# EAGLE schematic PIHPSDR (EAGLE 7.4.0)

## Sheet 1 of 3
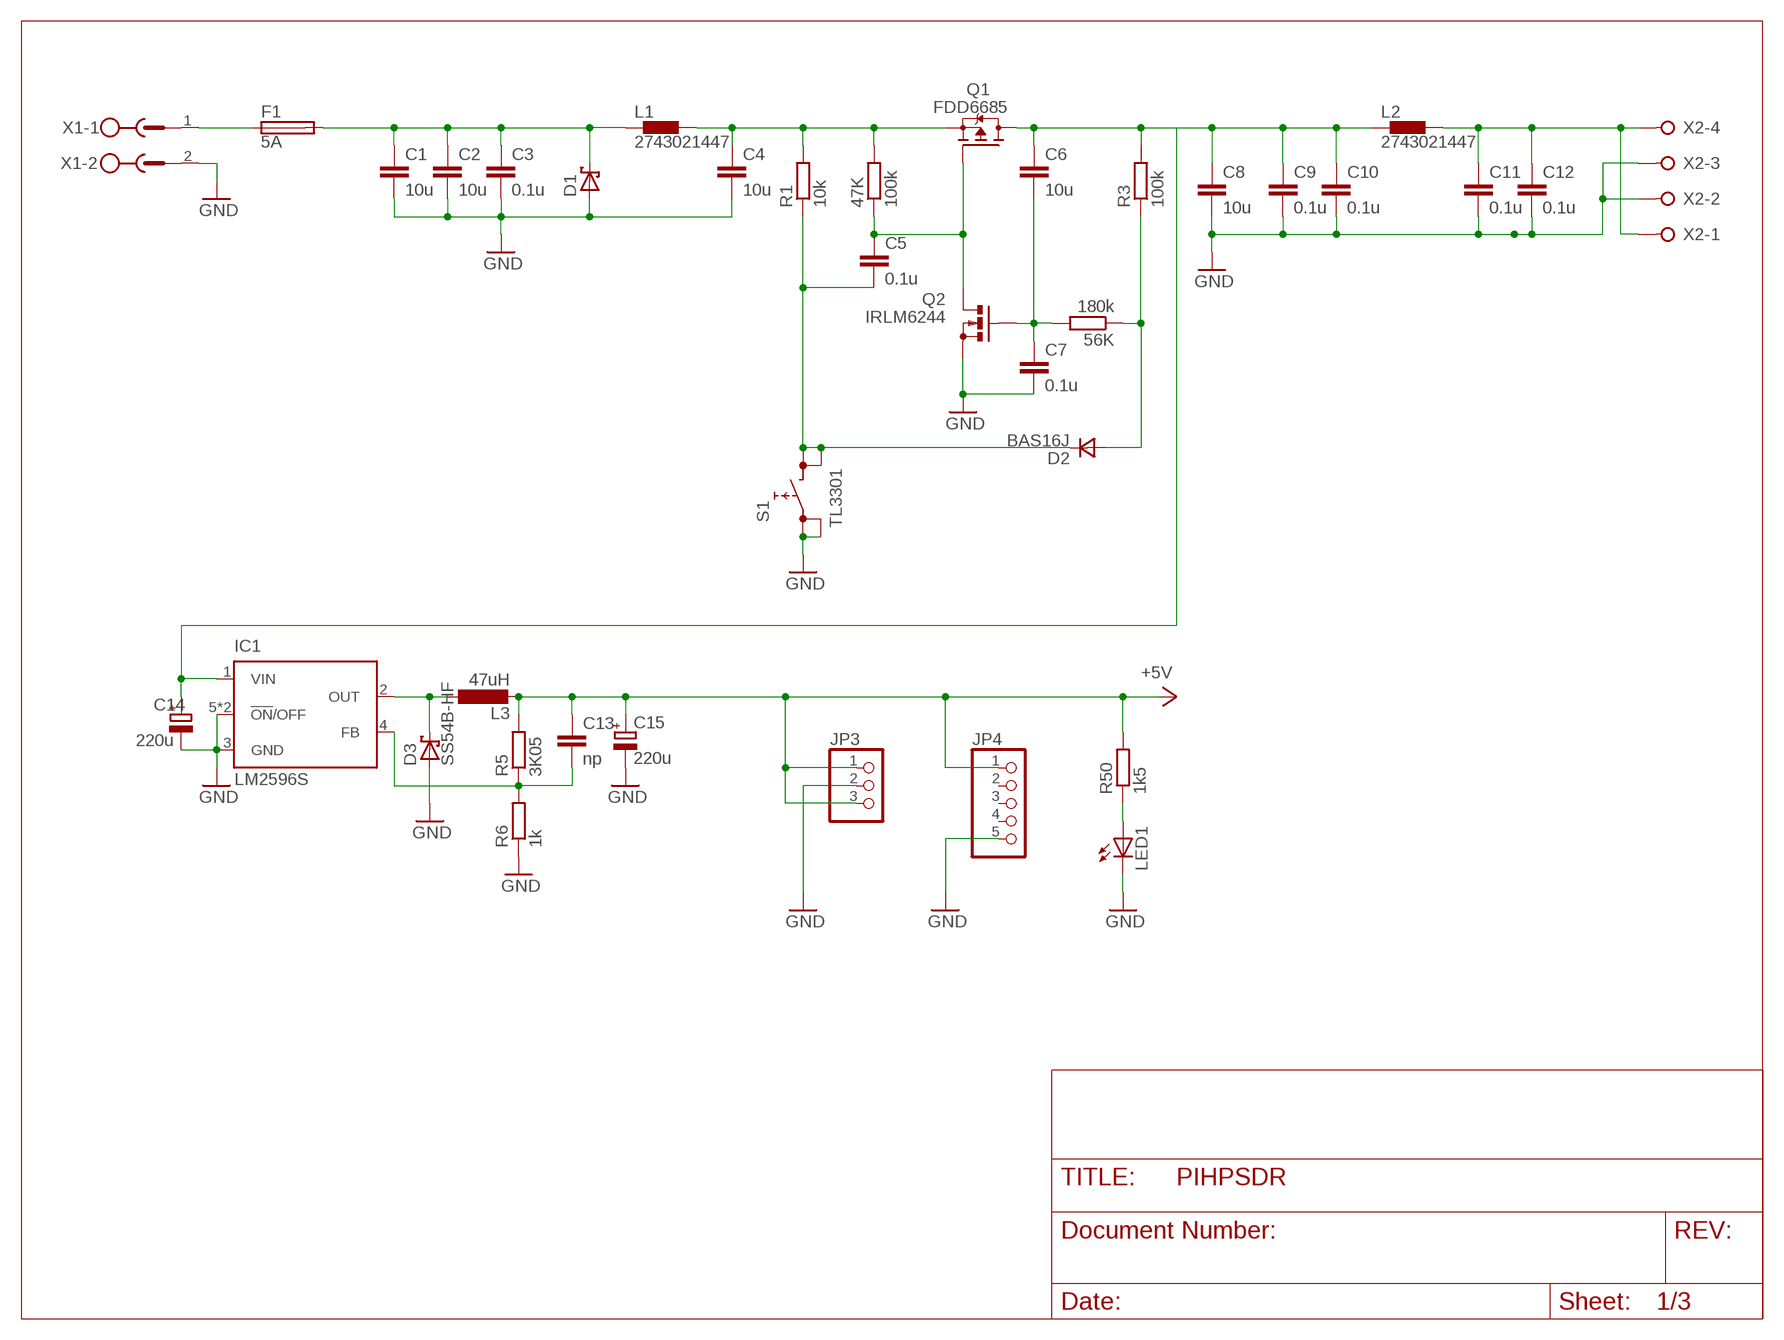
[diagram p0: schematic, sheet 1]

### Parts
47K  100k  R-EU_R0805  [R0805]
56K  180k  R-EU_R0805  [R0805]
C1  10u  C-EUC0805K  [C0805K]
C2  10u  C-EUC0805K  [C0805K]
C3  0.1u  C-EUC0805K  [C0805K]
C4  10u  C-EUC0805K  [C0805K]
C5  0.1u  C-EUC0805K  [C0805K]
C6  10u  C-EUC0805K  [C0805K]
C7  0.1u  C-EUC0805K  [C0805K]
C8  10u  C-EUC0805K  [C0805K]
C9  0.1u  C-EUC0805K  [C0805K]
C10  0.1u  C-EUC0805K  [C0805K]
C11  0.1u  C-EUC0805K  [C0805K]
C12  0.1u  C-EUC0805K  [C0805K]
C13  np  C-EUC0805  [C0805]
C14  220u  CPOL-EU140CLH-1010  [140CLH-1010]
C15  220u  CPOL-EU140CLH-1010  [140CLH-1010]
D1  SCHOTTKY-DIODESMC  [SMC]
D2  BAS16J  DSOD323  [SOD323]
D3  SS54B-HF  SCHOTTKY-DIODESMD  [SMB]
F1  5A  FUSESHK20L  [SHK20L]
IC1  LM2596S  [TO263-5]
JP3  PINHD-1X3  [1X03]
JP4  PINHD-1X5  [1X05]
L1  2743021447  [SM_BEAD]
L2  2743021447  [SM_BEAD]
L3  47uH  PULSE_PA4342  [PULSE_PA4342]
LED1  LED5MM  [LED5MM]
Q1  FDD6685  FDD4141TO252  [TO252]
Q2  IRLM6244  BS170_SMD  [SOT23]
R1  10k  R-EU_R0805  [R0805]
R3  100k  R-EU_R0805  [R0805]
R5  3K05  R-EU_R0805  [R0805]
R6  1k  R-EU_R0805  [R0805]
R50  1k5  R-EU_R0805  [R0805]
S1  TL3301  [TL3301-SMD]
X1  MSTBV2  [MSTBV2]
X2  W237-04P  [W237-4P]

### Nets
+5V: C13.1 C15.+ JP3.1 JP3.3 JP4.1 L3.2 R5.2 R50.2 ; also sheet 2,3
GND: C1.2 C2.2 C3.2 C4.2 C7.2 C8.2 C9.2 C10.2 C11.2 C12.2 C14.- C15.- D1.A D3.A IC1.3(GND) IC1.5(!ON!/OFF) IC1.6(!ON!/OFF) JP3.2 JP4.5 LED1.K(C) Q2.2(S) R6.1 S1.1 S1.2 X1.2 X2.2 X2.3 ; also sheet 2,3
N$1: F1.1A X1.1
N$2: C1.1 C2.1 C3.1 D1.C F1.2A L1.P$1
N$3: 47K.2 C4.1 L1.P$2 Q1.2(S) R1.2
N$4: 47K.1 C5.1 Q1.1(G) Q2.3(D)
N$5: C6.1 C8.1 C9.1 C10.1 C14.+ IC1.1(VIN) L2.P$1 Q1.3(D) R3.2
N$6: C5.2 D2.1(C) R1.1 S1.3 S1.4
N$7: 56K.2 C6.2 C7.1 Q2.1(G)
N$8: 56K.1 D2.2(A) R3.1
N$9: C11.1 C12.1 L2.P$2 X2.1 X2.4
N$10: D3.C IC1.2(OUT) L3.1
N$11: C13.2 IC1.4(FB) R5.1 R6.2
N$14: LED1.A R50.1
Unconnected: JP4.2 JP4.3 JP4.4

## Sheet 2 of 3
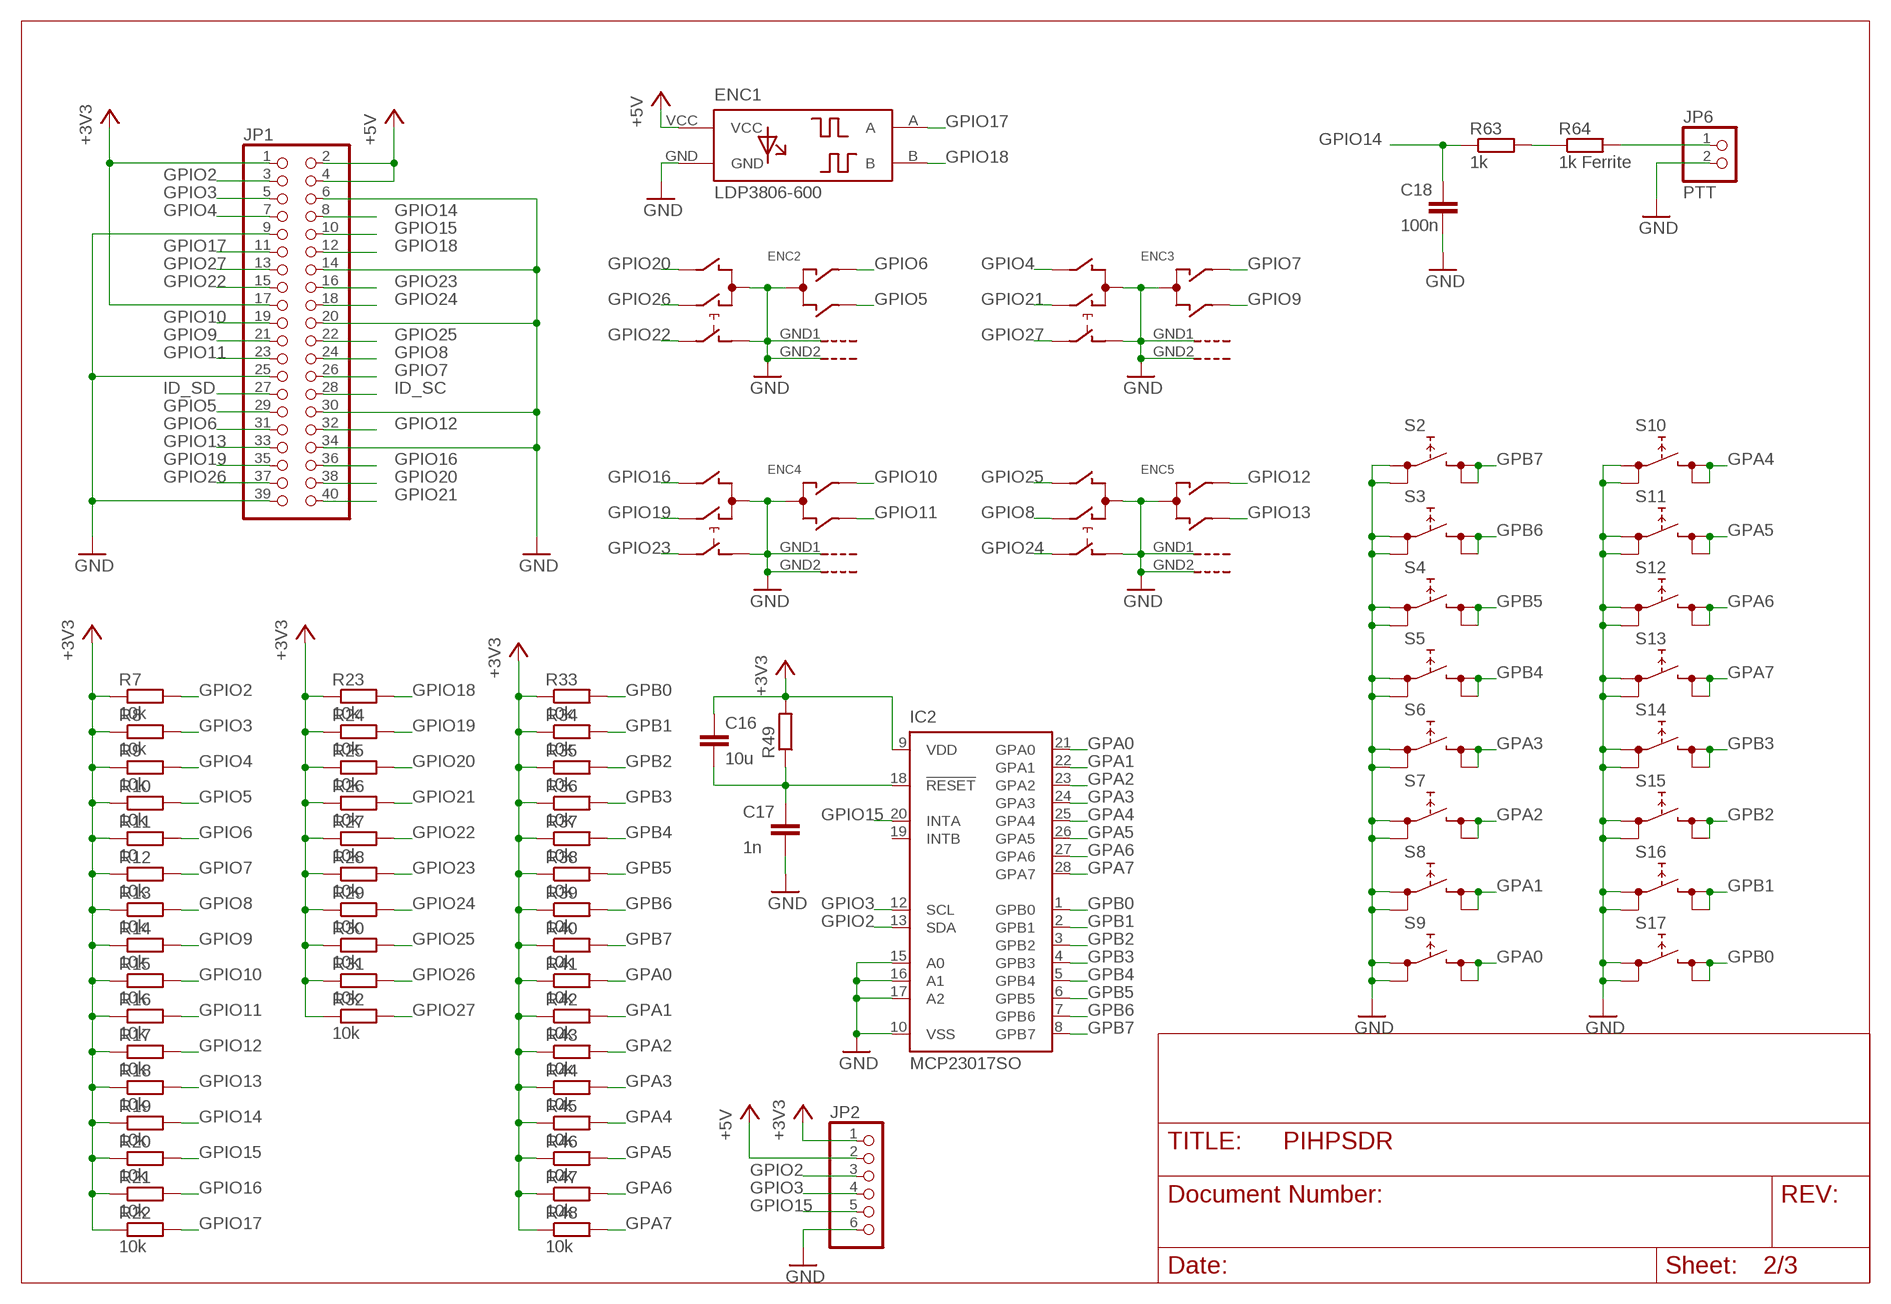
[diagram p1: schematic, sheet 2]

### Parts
C16  10u  C-EUC0805K  [C0805K]
C17  1n  C-EUC0805K  [C0805K]
C18  100n  C-EUC0805K  [C0805K]
ENC1  LDP3806-600  [LPD3806_ROTARY]
ENC2  EC11E_SW  [ALPS_EC11E_SW]
ENC3  EC11E_SW  [ALPS_EC11E_SW]
ENC4  EC11E_SW  [ALPS_EC11E_SW]
ENC5  EC11E_SW  [ALPS_EC11E_SW]
IC2  MCP23017SO  [SO28W]
JP1  PINHD-2X20  [2X20]
JP2  PINHD-1X6  [1X06]
JP6  PTT  PINHD-1X2  [1X02]
R7  10k  R-EU_R0805  [R0805]
R8  10k  R-EU_R0805  [R0805]
R9  10k  R-EU_R0805  [R0805]
R10  10k  R-EU_R0805  [R0805]
R11  10  R-EU_R0805  [R0805]
R12  10k  R-EU_R0805  [R0805]
R13  10k  R-EU_R0805  [R0805]
R14  10k  R-EU_R0805  [R0805]
R15  10k  R-EU_R0805  [R0805]
R16  10k  R-EU_R0805  [R0805]
R17  10k  R-EU_R0805  [R0805]
R18  10k  R-EU_R0805  [R0805]
R19  10k  R-EU_R0805  [R0805]
R20  10k  R-EU_R0805  [R0805]
R21  10k  R-EU_R0805  [R0805]
R22  10k  R-EU_R0805  [R0805]
R23  10k  R-EU_R0805  [R0805]
R24  10k  R-EU_R0805  [R0805]
R25  10k  R-EU_R0805  [R0805]
R26  10k  R-EU_R0805  [R0805]
R27  10k  R-EU_R0805  [R0805]
R28  10k  R-EU_R0805  [R0805]
R29  10k  R-EU_R0805  [R0805]
R30  10k  R-EU_R0805  [R0805]
R31  10k  R-EU_R0805  [R0805]
R32  10k  R-EU_R0805  [R0805]
R33  10k  R-EU_R0805  [R0805]
R34  10k  R-EU_R0805  [R0805]
R35  10k  R-EU_R0805  [R0805]
R36  10k  R-EU_R0805  [R0805]
R37  10k  R-EU_R0805  [R0805]
R38  10k  R-EU_R0805  [R0805]
R39  10k  R-EU_R0805  [R0805]
R40  10k  R-EU_R0805  [R0805]
R41  10k  R-EU_R0805  [R0805]
R42  10k  R-EU_R0805  [R0805]
R43  10k  R-EU_R0805  [R0805]
R44  10k  R-EU_R0805  [R0805]
R45  10k  R-EU_R0805  [R0805]
R46  10k  R-EU_R0805  [R0805]
R47  10k  R-EU_R0805  [R0805]
R48  10k  R-EU_R0805  [R0805]
R49  R-EU_R0805  [R0805]
R63  1k  R-EU_R0805  [R0805]
R64  1k Ferrite  R-EU_R0805  [R0805]
S2  TL3301  [TL3301-SMD]
S3  TL3301  [TL3301-SMD]
S4  TL3301  [TL3301-SMD]
S5  TL3301  [TL3301-SMD]
S6  TL3301  [TL3301-SMD]
S7  TL3301  [TL3301-SMD]
S8  TL3301  [TL3301-SMD]
S9  TL3301  [TL3301-SMD]
S10  TL3301  [TL3301-SMD]
S11  TL3301  [TL3301-SMD]
S12  TL3301  [TL3301-SMD]
S13  TL3301  [TL3301-SMD]
S14  TL3301  [TL3301-SMD]
S15  TL3301  [TL3301-SMD]
S16  TL3301  [TL3301-SMD]
S17  TL3301  [TL3301-SMD]

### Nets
+3V3: C16.1 IC2.9(VDD) JP1.1 JP1.17 JP2.1 R7.1 R8.1 R9.1 R10.1 R11.1 R12.1 R13.1 R14.1 R15.1 R16.1 R17.1 R18.1 R19.1 R20.1 R21.1 R22.1 R23.1 R24.1 R25.1 R26.1 R27.1 R28.1 R29.1 R30.1 R31.1 R32.1 R33.1 R34.1 R35.1 R36.1 R37.1 R38.1 R39.1 R40.1 R41.1 R42.1 R43.1 R44.1 R45.1 R46.1 R47.1 R48.1 R49.2
+5V: ENC1.VCC JP1.2 JP1.4 JP2.2 ; also sheet 1,3
GND: C17.2 C18.2 ENC1.GND ENC2.C ENC2.C'(C) ENC2.D ENC2.GND1(G) ENC2.GND2(G) ENC3.C ENC3.C'(C) ENC3.D ENC3.GND1(G) ENC3.GND2(G) ENC4.C ENC4.C'(C) ENC4.D ENC4.GND1(G) ENC4.GND2(G) ENC5.C ENC5.C'(C) ENC5.D ENC5.GND1(G) ENC5.GND2(G) IC2.10(VSS) IC2.15(A0) IC2.16(A1) IC2.17(A2) JP1.6 JP1.9 JP1.14 JP1.20 JP1.25 JP1.30 JP1.34 JP1.39 JP2.6 JP6.2 S2.1 S2.2 S3.1 S3.2 S4.1 S4.2 S5.1 S5.2 S6.1 S6.2 S7.1 S7.2 S8.1 S8.2 S9.1 S9.2 S10.1 S10.2 S11.1 S11.2 S12.1 S12.2 S13.1 S13.2 S14.1 S14.2 S15.1 S15.2 S16.1 S16.2 S17.1 S17.2 ; also sheet 1,3
GPA0: IC2.21(GPA0) R41.2 S9.3 S9.4
GPA1: IC2.22(GPA1) R42.2 S8.3 S8.4
GPA2: IC2.23(GPA2) R43.2 S7.3 S7.4
GPA3: IC2.24(GPA3) R44.2 S6.3 S6.4
GPA4: IC2.25(GPA4) R45.2 S10.3 S10.4
GPA5: IC2.26(GPA5) R46.2 S11.3 S11.4
GPA6: IC2.27(GPA6) R47.2 S12.3 S12.4
GPA7: IC2.28(GPA7) R48.2 S13.3 S13.4
GPB0: IC2.1(GPB0) R33.2 S17.3 S17.4
GPB1: IC2.2(GPB1) R34.2 S16.3 S16.4
GPB2: IC2.3(GPB2) R35.2 S15.3 S15.4
GPB3: IC2.4(GPB3) R36.2 S14.3 S14.4
GPB4: IC2.5(GPB4) R37.2 S5.3 S5.4
GPB5: IC2.6(GPB5) R38.2 S4.3 S4.4
GPB6: IC2.7(GPB6) R39.2 S3.3 S3.4
GPB7: IC2.8(GPB7) R40.2 S2.3 S2.4
GPIO2: IC2.13(SDA) JP1.3 JP2.3 R7.2
GPIO3: IC2.12(SCL) JP1.5 JP2.4 R8.2
GPIO4: ENC3.B JP1.7 R9.2
GPIO5: ENC2.B'(B) JP1.29 R10.2
GPIO6: ENC2.A'(A) JP1.31 R11.2
GPIO7: ENC3.A'(A) JP1.26 R12.2
GPIO8: ENC5.A JP1.24 R13.2
GPIO9: ENC3.B'(B) JP1.21 R14.2
GPIO10: ENC4.A'(A) JP1.19 R15.2
GPIO11: ENC4.B'(B) JP1.23 R16.2
GPIO12: ENC5.A'(A) JP1.32 R17.2
GPIO13: ENC5.B'(B) JP1.33 R18.2
GPIO14: C18.1 JP1.8 R19.2 R63.1
GPIO15: IC2.20(INTA) JP1.10 JP2.5 R20.2
GPIO16: ENC4.B JP1.36 R21.2
GPIO17: ENC1.A JP1.11 R22.2
GPIO18: ENC1.B JP1.12 R23.2
GPIO19: ENC4.A JP1.35 R24.2
GPIO20: ENC2.B JP1.38 R25.2
GPIO21: ENC3.A JP1.40 R26.2
GPIO22: ENC2.E JP1.15 R27.2
GPIO23: ENC4.E JP1.16 R28.2
GPIO24: ENC5.E JP1.18 R29.2
GPIO25: ENC5.B JP1.22 R30.2
GPIO26: ENC2.A JP1.37 R31.2
GPIO27: ENC3.E JP1.13 R32.2
ID_SC: JP1.28
ID_SD: JP1.27
N$12: C16.2 C17.1 IC2.18(!RESET) R49.1
N$32: R63.2 R64.1
N$33: JP6.1 R64.2
Unconnected: IC2.19(INTB)

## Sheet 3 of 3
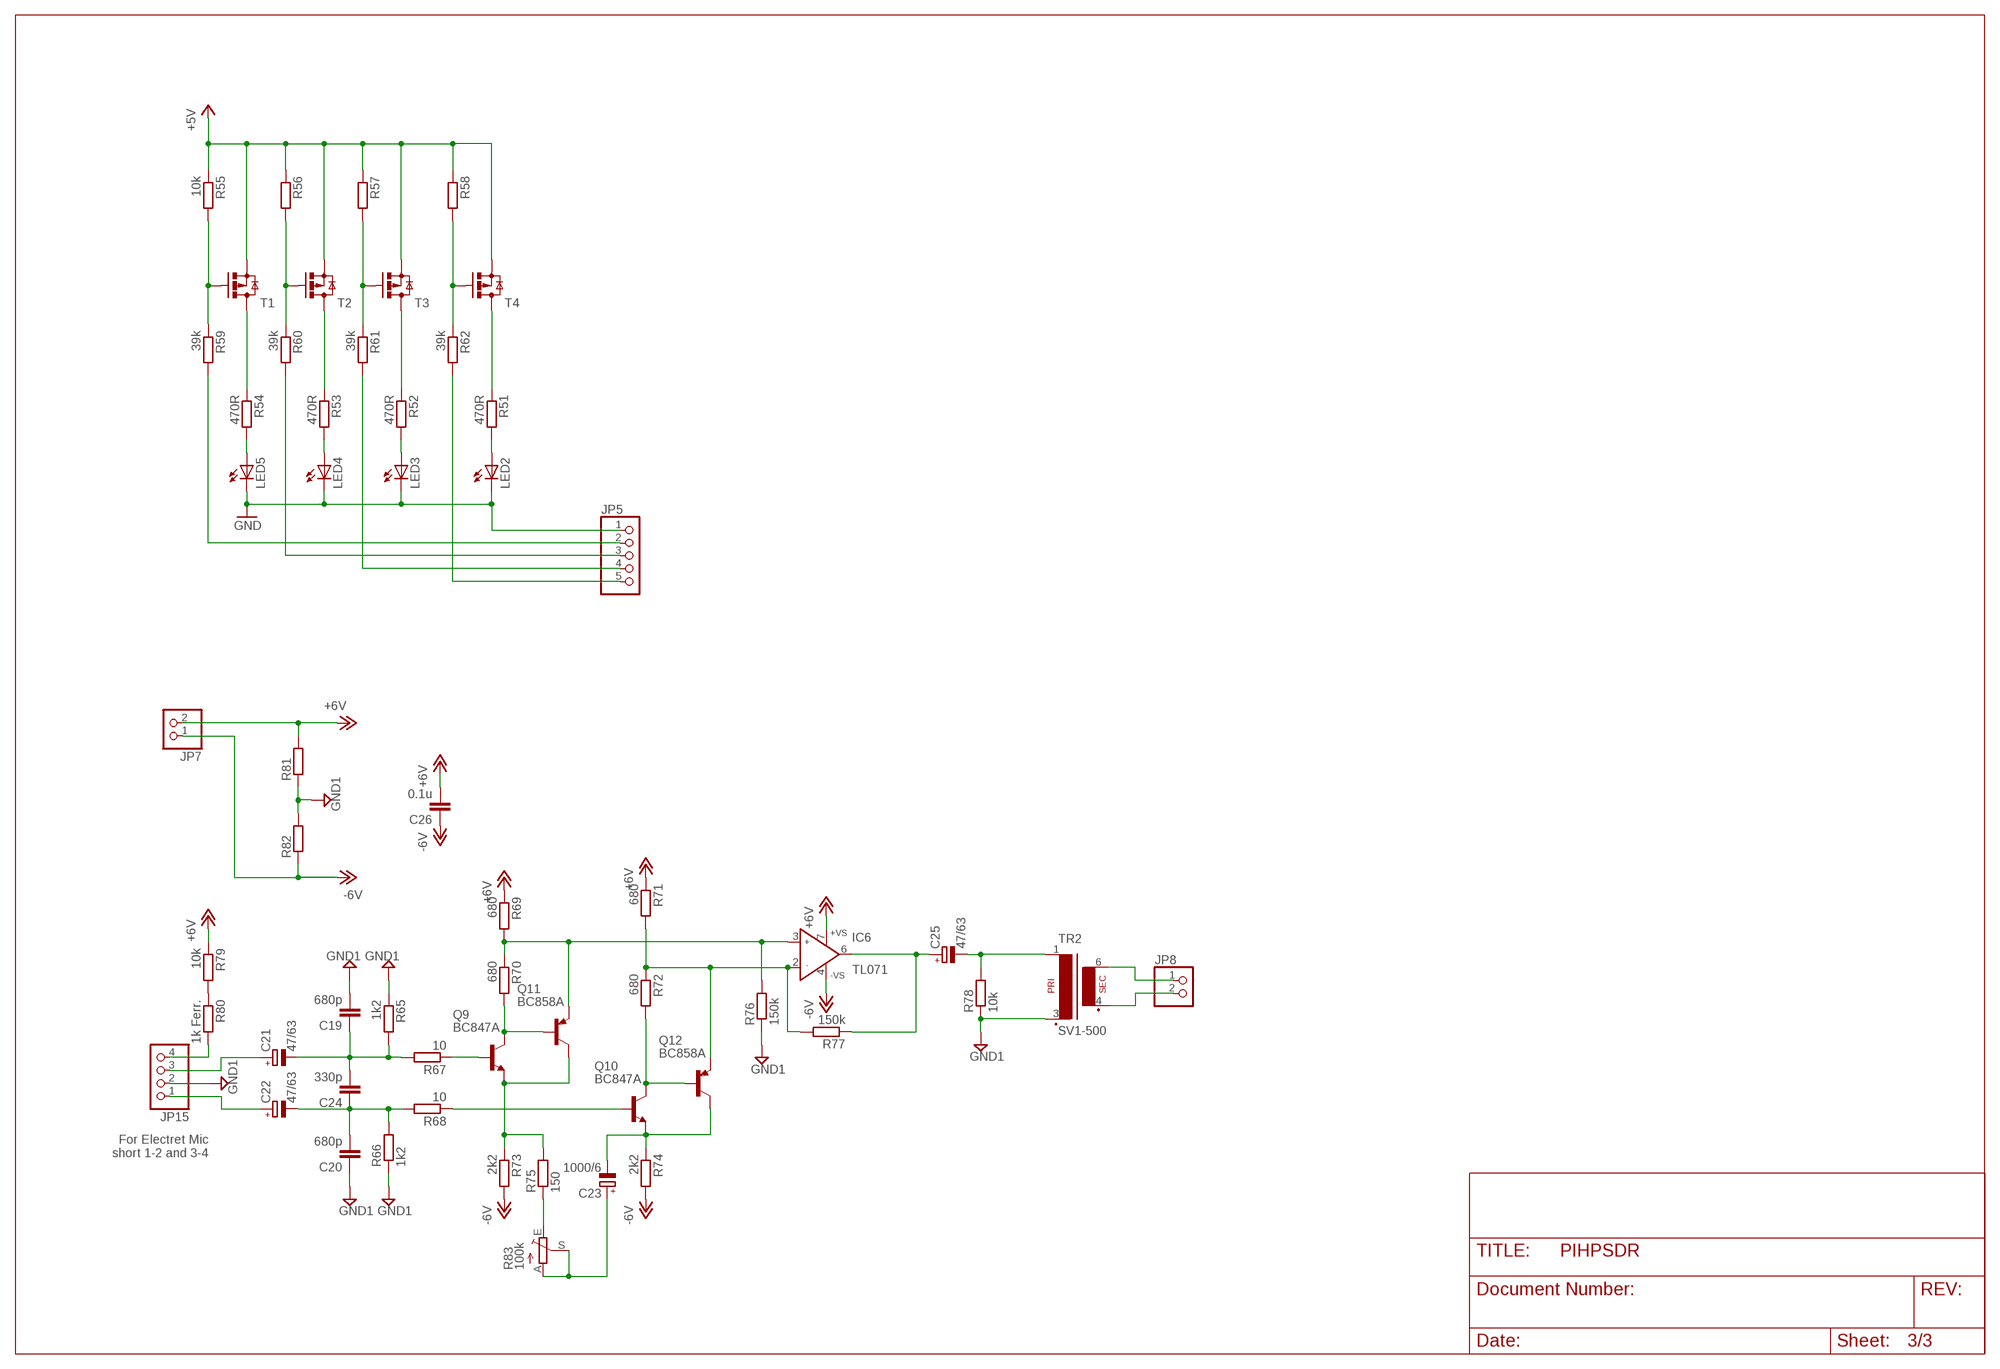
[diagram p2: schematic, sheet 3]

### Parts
C19  680p  C-EUC0805  [C0805]
C20  680p  C-EUC0805  [C0805]
C21  47/63  CPOL-EUE2.5-7  [E2,5-7]
C22  47/63  CPOL-EUE2.5-7  [E2,5-7]
C23  1000/6  CPOL-EUE5-10.5  [E5-10,5]
C24  330p  C-EUC0805  [C0805]
C25  47/63  CPOL-EUE2.5-7  [E2,5-7]
C26  0.1u  C-EUC0805  [C0805]
IC6  TL071  AD820R  [SO8]
JP5  PINHD-1X5  [1X05]
JP7  PINHD-1X2  [1X02]
JP8  PINHD-1X2  [1X02]
JP15  PINHD-1X4  [1X04]
LED2  LED5MM  [LED5MM]
LED3  LED5MM  [LED5MM]
LED4  LED5MM  [LED5MM]
LED5  LED5MM  [LED5MM]
Q9  BC847A  BC847ASMD  [SOT23]
Q10  BC847A  BC847ASMD  [SOT23]
Q11  BC858A  BC858ASMD  [SOT23-BEC]
Q12  BC858A  BC858ASMD  [SOT23-BEC]
R51  470R  R-EU_R0805  [R0805]
R52  470R  R-EU_R0805  [R0805]
R53  470R  R-EU_R0805  [R0805]
R54  470R  R-EU_R0805  [R0805]
R55  10k  R-EU_R0805  [R0805]
R56  R-EU_R0805  [R0805]
R57  R-EU_R0805  [R0805]
R58  R-EU_R0805  [R0805]
R59  39k  R-EU_R0805  [R0805]
R60  39k  R-EU_R0805  [R0805]
R61  39k  R-EU_R0805  [R0805]
R62  39k  R-EU_R0805  [R0805]
R65  1k2  R-EU_R0805  [R0805]
R66  1k2  R-EU_R0805  [R0805]
R67  10  R-EU_R0805  [R0805]
R68  10  R-EU_R0805  [R0805]
R69  680  R-EU_R0805  [R0805]
R70  680  R-EU_R0805  [R0805]
R71  680  R-EU_R0805  [R0805]
R72  680  R-EU_R0805  [R0805]
R73  2k2  R-EU_R0805  [R0805]
R74  2k2  R-EU_R0805  [R0805]
R75  150  R-EU_R0805  [R0805]
R76  150k  R-EU_R0805  [R0805]
R77  150k  R-EU_R0805  [R0805]
R78  10k  R-EU_R0805  [R0805]
R79  10k  R-EU_R0805  [R0805]
R80  1k Ferr.  R-EU_R0805  [R0805]
R81  R-EU_0207/10  [0207/10]
R82  R-EU_0207/10  [0207/10]
R83  100k  TRIM_EU-S64W  [S64W]
T1  DMP2045U  [SOT23]
T2  DMP2045U  [SOT23]
T3  DMP2045U  [SOT23]
T4  DMP2045U  [SOT23]
TR2  SV1-500  [SV1-500]

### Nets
+5V: R55.1 R56.1 R57.1 R58.1 T1.2(S) T2.2(S) T3.2(S) T4.2(S) ; also sheet 1,2
+12V: C26.2 IC6.7(+VS) JP7.2 R69.1 R71.1 R79.1 R81.2 ; supply symbol labelled +6V
-12V: C26.1 IC6.4(-VS) JP7.1 R73.2 R74.2 R82.1 ; supply symbol labelled -6V
GND: JP5.1 LED2.K(C) LED3.K(C) LED4.K(C) LED5.K(C) ; also sheet 1,2
GND1: C19.2 C20.1 JP15.2 R65.1 R66.1 R76.1 R78.1 R81.1 R82.2 TR2.3(P2)
N$13: R55.2 R59.1 T1.1(G)
N$15: R56.2 R60.1 T2.1(G)
N$16: LED2.A R51.2
N$17: LED3.A R52.2
N$18: LED4.A R53.2
N$19: LED5.A R54.2
N$20: R57.2 R61.1 T3.1(G)
N$21: R58.2 R62.1 T4.1(G)
N$22: R54.1 T1.3(D)
N$23: JP5.2 R59.2
N$24: JP5.3 R60.2
N$25: JP5.4 R61.2
N$26: JP5.5 R62.2
N$27: R53.1 T2.3(D)
N$28: R52.1 T3.3(D)
N$29: R51.1 T4.3(D)
N$30: JP8.1 TR2.6(S4)
N$31: JP8.2 TR2.4(S3)
N$34: R75.1 R83.E
N$35: C23.+ R83.A R83.S
N$96: Q9.3(C) Q11.B R70.2
N$97: IC6.3(IN+) Q11.E R69.2 R70.1 R76.2
N$98: C20.2 C22.- C24.1 R66.2 R68.2
N$99: Q9.2(E) Q11.C R73.1 R75.2
N$100: Q9.1(B) R67.1
N$101: C19.1 C21.- C24.2 R65.2 R67.2
N$102: Q10.1(B) R68.1
N$103: IC6.2(IN-) Q12.E R71.2 R72.1 R77.2
N$104: Q10.3(C) Q12.B R72.2
N$105: C23.- Q10.2(E) Q12.C R74.1
N$107: C25.+ IC6.6(OUT) R77.1
N$110: C21.+ JP15.3
N$111: C22.+ JP15.1
N$112: C25.- R78.2 TR2.1
N$149: R79.2 R80.1
N$150: JP15.4 R80.2

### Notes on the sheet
- For Electret Mic
  short 1-2 and 3-4

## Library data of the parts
47K 56K R1 R3 R5-R82 = rcl:R-EU_: RESISTOR, European symbol
C1-C13 C16-C20 C24 C26 = rcl:C-EU: CAPACITOR, European symbol
C14 C15 C21-C23 C25 = rcl:CPOL-EU: POLARIZED CAPACITOR, European symbol
D1 D3 = diode:SCHOTTKY-DIODE: Schottky Diode
D2 = zetex:D: DIODE; MPN: CDSOD323-T05C; OC_FARNELL: 1824860; OC_NEWARK: 79R6078
ENC1 = HM:LDP3806-600: 360/600P/R Photoelectric Incremental Rotary Encoder 5V-24V AB Two Phases Shaft F
ENC2-ENC5 = switch-alps:EC11E_SW: Dual-shaft type with push-on switch （travel 1.5mm） Inner shaft: encoder Outer shaft: self-return switch
F1 = fuse:FUSE: Fuse; OC_FARNELL: unknown; OC_NEWARK: unknown
IC1 = national-semiconductor:LM2596: SIMPLE SWITCHER® Power Converter 150 kHz 3A Step-Down Voltage Regulator Source: http://www.national.com/ds/LM/LM2596.pdf; MF: NATIONAL SEMICONDUCTOR; MPN: LM2596S-ADJ/NOPB; OC_FARNELL: 9494367; OC_NEWARK: 41K3842
IC2 = microchip:MCP23017: http://ww1.microchip.com/downloads/en/DeviceDoc/21952a.pdf Source: http://ww1.microchip.com/downloads/en/DeviceDoc/21952a.pdf; MF: MICROCHIP; MPN: MCP23017-E/SO; OC_FARNELL: 1332087; OC_NEWARK: 31K2958
IC6 = analog-devices:AD820: Single-Supply, Rail-to-Rail, Low Power, FET Input Op Amp Source: http://www.analog.com/static/imported-files/data_sheets/AD820.pdf; OC_FARNELL: 1838867; OC_NEWARK: unknown
JP1 = pinhead:PINHD-2X20: PIN HEADER
JP2 = pinhead:PINHD-1X6: PIN HEADER
JP3 = pinhead:PINHD-1X3: PIN HEADER
JP4 JP5 = pinhead:PINHD-1X5: PIN HEADER
JP6-JP8 = pinhead:PINHD-1X2: PIN HEADER
JP15 = pinhead:PINHD-1X4: PIN HEADER
L1 L2 = inductors:2743021447: Ferrite Beads 43 SM BEAD Z=95 OHM @100MHz
L3 = rcl:PULSE_PA4342: PULSE PA4342 SMD inductor
LED1-LED5 = led:LED: LED
Q1 = transistor-fet:FDD4141: P-Channel PowerTrench® MOSFET Source: FDD4141.pdf
Q2 = HM:BS170_: N-CHANNEL MOS FET
Q9 Q10 = transistor-npn:BC847*: NPN Transistor
Q11 Q12 = transistor-pnp:BC858*: PNP Transistror
R83 = pot:TRIM_EU-: POTENTIOMETER
S1-S17 = switch:TL3301: 6 x 6mm TACT Switch (SMD)
T1-T4 = HM:DMP2045U: P-MOSFET SOT32
TR2 = Mic-ControllerV2:SV1-500: Audio Transfomer
X1 = con-phoenix-500:MSTBV2: PHOENIX; OC_FARNELL: unknown; OC_NEWARK: unknown
X2 = con-wago-508:W237-04P: WAGO SREW CLAMP; OC_FARNELL: unknown; OC_NEWARK: unknown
